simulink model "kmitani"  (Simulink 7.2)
settings: Solver=ode45  StartTime=0.0  StopTime=50  RelTol=1e-3
InitFcn:
  | init_kmitani;
StopFcn:
  | post;
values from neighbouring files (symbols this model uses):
  amp = 5    [init_kmitani.m]
  freq = 50.2248    [init_kmitani.m]
  I_tycka = (m_tycka*l_tycka^2)/12 * [0 0 0;0 1 0; 0 0 1]    [init_kmitani.m]
  I_zavazi = [(m_zavazi/4)*(R_zavazi^2 + (h_zavazi^2)/3 ) 0 0    [init_kmitani.m]
  l_tycka = 1    [init_kmitani.m]
  m = 1    [smykadlo_init.m]
  m_tycka = 0.001    [init_kmitani.m]
  m_zavazi = 10    [init_kmitani.m]
  R_zavazi = 0.1    [init_kmitani.m]
  vule_H = 0.01    [init_kmitani.m]
  vule_L = -0.18    [init_kmitani.m]
undefined symbols (not defined in the file or in its folder): deg, kg, N, s
libraries: mblibv1 x13

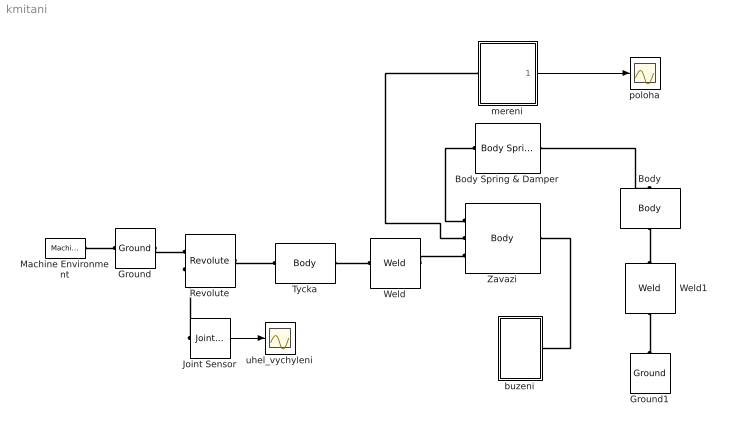
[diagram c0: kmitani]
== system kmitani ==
  Body : mblibv1/Bodies/Body  Orientation=up  DialogController=MECH.DynMechDlgSource  PhysicalDomain=mechanical  SubClassName=Unknown  LeftPortType=workingframe  RightPortType=workingframe  LConnTagsString=CS1  RConnTagsString=CS2  UpdateFromCAD=off  DialogClass=MechanicalBodyBlock  Mass=0  MassUnits=kg  InertiaUnits=kg*m^2  Inertia=zeros(3)  Shape=Cylinder  ShapeDims=[1 1]  ShapeUnits=m  ShapeUse=false  Density=1  DensityUnits=kg/m^3  DensityUse=false  GraphicsMode=MACHINE_DEFAULT  BodyColorSelMode=MACHINE_DEFAULT  BodyColor=[1 0 0]  AttachedToCS=CG  CG=Left$CG$[0 0 0]$CS1$CS1$m$[0 0 0]$Euler X-Y-Z$deg$WORLD$false$none  WorkingFrames=Left$CS1$[0 0 0]$Adjoining$Adjoining$m$[0 0 0]$Euler X-Y-Z$deg$WORLD$true$none#Right$CS2$[0 0 0]$CS1$CS1$m$[0 0 0]$Euler X-Y-Z$deg$WORLD$true$none  CGPos=[0 0 0]  CGRot=[0 0 0]  CS0Pos=[]  CS0Rot=[]  CS1Pos=[0 0 0]  CS1Rot=[0 0 0]  CS2Pos=[0 0 0]  CS2Rot=[0 0 0]  CS3Pos=[]  CS3Rot=[]  CS4Pos=[]  CS4Rot=[]  CS5Pos=[]  CS5Rot=[]  CS6Pos=[]  CS6Rot=[]  CS7Pos=[]  CS7Rot=[]  CS8Pos=[]  CS8Rot=[]  CS9Pos=[]  CS9Rot=[]  CS10Pos=[]  CS10Rot=[]  CS11Pos=[]  CS11Rot=[]  CS12Pos=[]  CS12Rot=[]  CS13Pos=[]  CS13Rot=[]  CS14Pos=[]  CS14Rot=[]  CS15Pos=[]  CS15Rot=[]  CS16Pos=[]  CS16Rot=[]  CS17Pos=[]  CS17Rot=[]  CS18Pos=[]  CS18Rot=[]  CS19Pos=[]  CS19Rot=[]  CS20Pos=[]  CS20Rot=[]
  Body Spring & Damper : mblibv1/Force  Elements/Body Spring & Damper  DialogController=MECH.DynMechDlgSource  SystemSampleTime=-1  UpdateFromCAD=off  DialogClass=BodySpringDamper  Spring_k=k  Damper_b=b  Offset_x0=0  PositionUnits=m  VelocityUnits=m/s  ForceUnits=N
  Ground : mblibv1/Bodies/Ground  DialogController=MECH.DynMechDlgSource  SystemSampleTime=-1  UpdateFromCAD=off  LeftPortType=env  RightPortType=workingframe  PhysicalDomain=Mechanical  DialogClass=GroundBlock  CoordPosition=[0 0 0]  CoordPositionUnits=m  StateVectorMgrId=-1  MachineId=[0 0]  ShowEnvPort=on
  Ground1 : mblibv1/Bodies/Ground  Orientation=up  DialogController=MECH.DynMechDlgSource  SystemSampleTime=-1  UpdateFromCAD=off  LeftPortType=env  RightPortType=workingframe  PhysicalDomain=Mechanical  DialogClass=GroundBlock  CoordPosition=[l_tycka+R_zavazi 0 0]  CoordPositionUnits=m  StateVectorMgrId=-1  MachineId=[0 0]  ShowEnvPort=off
  Joint Sensor : mblibv1/Sensors &  Actuators/Joint Sensor  DialogController=MECH.DynMechDlgSource  SystemSampleTime=-1  UpdateFromCAD=off  PhysicalDomain=Mechanical  PortType=blob  Muxed=on  Pose=off  Angle=on  AngleUnits=rad  ArcVelocity=off  ArcVelocityUnits=deg/s  ArcAcceleration=off  ArcAccelerationUnits=deg/s^2  CoordPosition=on  CoordPositionUnits=m  Velocity=off  VelocityUnits=m/s  Acceleration=off  AccelerationUnits=m/s^2  Quaternion=on  QuaternionDT=off  QuaternionDDT=off  QuaternionUnits=off  OutputVector=[1]  ActiveIO=off  Width=1  DialogClass=MechanicalSensorBlock  Primitive=R1  Force=off  ForceUnits=N  Torque=off  TorqueUnits=N*m  ReferenceFrame=Absolute (World)  ReactionSensedSide=Base  ReactionReferenceFrame=Absolute (World)  ReactionForce=off  ReactionForceUnits=N  ReactionMoment=off  ReactionMomentUnits=N*m
  Machine Environment : mblibv1/Bodies/Machine Environment  DialogController=MECH.DialogSource  SystemSampleTime=-1  PortType=env  PhysicalDomain=Mechanical  DialogTemplateClass=MECH.MachineEnvironment  SyncWhenCopied=off  Gravity=[0 0 0]  GravityUnits=m/s^2  GravityAsSignal=off  Dimensionality=Auto-detect  AnalysisType=Forward dynamics  LinearAssemblyTolerance=1e-3  LinearAssemblyToleranceUnits=m  AngularAssemblyTolerance=1e-3  AngularAssemblyToleranceUnits=rad  ConstraintSolverType=Stabilizing  ConstraintRelTolerance=1e-4  ConstraintAbsTolerance=1e-4  UseRobustSingularityHandling=off  RedundancyAnalysisToleranceType=Automatically select tolerance  RedundancyAnalysisTolerance=1e-14  StatePerturbationType=Fixed  PerturbationSize=1e-5  VisualizeMachine=on  BodyVisualizationType=Use model default body geometries  BodyColorSelMode=Use model default  DefaultBodyColor=[1 0 0]
  Revolute : mblibv1/Joints/Revolute  DialogController=MECH.DynMechDlgSource  PhysicalDomain=mechanical  SubClassName=Unknown  LeftPortType=blob  RightPortType=blob  LConnTagsString=__newl0|SA1  RConnTagsString=__newr0  UpdateFromCAD=off  NumSAPorts=1  CutJoint=off  MarkAsCut=off  Primitives=prismatic  PrimitiveProps=R1$World$[0 0 1]$revolute  DialogClass=JointBlock  R1Axis=[0 0 1]
  Tycka : mblibv1/Bodies/Body  DialogController=MECH.DynMechDlgSource  PhysicalDomain=mechanical  SubClassName=Unknown  LeftPortType=workingframe  RightPortType=workingframe  LConnTagsString=CS1  RConnTagsString=CS2  UpdateFromCAD=off  DialogClass=MechanicalBodyBlock  Mass=m_tycka  MassUnits=kg  InertiaUnits=kg*m^2  Inertia=I_tycka  Shape=Cylinder  ShapeDims=[1 1]  ShapeUnits=m  ShapeUse=false  Density=1  DensityUnits=kg/m^3  DensityUse=false  GraphicsMode=MACHINE_DEFAULT  BodyColorSelMode=MACHINE_DEFAULT  BodyColor=[1 0 0]  AttachedToCS=CG  CG=Left$CG$[l_tycka/2 0 0]$CS1$CS1$m$[0 0 0]$Euler X-Y-Z$deg$WORLD$false$none  WorkingFrames=Left$CS1$[0 0 0]$Adjoining$Adjoining$m$[0 0 0]$Euler X-Y-Z$deg$WORLD$true$none#Right$CS2$[l_tycka 0 0]$CS1$CS1$m$[0 0 0]$Euler X-Y-Z$deg$WORLD$true$none  CGPos=[l_tycka/2 0 0]  CGRot=[0 0 0]  CS0Pos=[]  CS0Rot=[]  CS1Pos=[0 0 0]  CS1Rot=[0 0 0]  CS2Pos=[l_tycka 0 0]  CS2Rot=[0 0 0]  CS3Pos=[]  CS3Rot=[]  CS4Pos=[]  CS4Rot=[]  CS5Pos=[]  CS5Rot=[]  CS6Pos=[]  CS6Rot=[]  CS7Pos=[]  CS7Rot=[]  CS8Pos=[]  CS8Rot=[]  CS9Pos=[]  CS9Rot=[]  CS10Pos=[]  CS10Rot=[]  CS11Pos=[]  CS11Rot=[]  CS12Pos=[]  CS12Rot=[]  CS13Pos=[]  CS13Rot=[]  CS14Pos=[]  CS14Rot=[]  CS15Pos=[]  CS15Rot=[]  CS16Pos=[]  CS16Rot=[]  CS17Pos=[]  CS17Rot=[]  CS18Pos=[]  CS18Rot=[]  CS19Pos=[]  CS19Rot=[]  CS20Pos=[]  CS20Rot=[]
  Weld : mblibv1/Joints/Weld  DialogController=MECH.DynMechDlgSource  PhysicalDomain=mechanical  SubClassName=Unknown  LeftPortType=blob  RightPortType=blob  LConnTagsString=__newl0  RConnTagsString=__newr0  UpdateFromCAD=off  NumSAPorts=0  CutJoint=off  MarkAsCut=off  Primitives=weld  PrimitiveProps=W$WORLD$[0 0 0]$weld  DialogClass=JointBlock  WAxis=[0 0 0]
  Weld1 : mblibv1/Joints/Weld  Orientation=up  DialogController=MECH.DynMechDlgSource  PhysicalDomain=mechanical  SubClassName=Unknown  LeftPortType=blob  RightPortType=blob  LConnTagsString=__newl0  RConnTagsString=__newr0  UpdateFromCAD=off  NumSAPorts=0  CutJoint=off  MarkAsCut=off  Primitives=weld  PrimitiveProps=W$WORLD$[0 0 0]$weld  DialogClass=JointBlock  WAxis=[0 0 0]
  Zavazi : mblibv1/Bodies/Body  DialogController=MECH.DynMechDlgSource  PhysicalDomain=mechanical  SubClassName=Unknown  LeftPortType=workingframe  RightPortType=workingframe  LConnTagsString=CG|CS5|CS1  RConnTagsString=CS2  UpdateFromCAD=off  DialogClass=MechanicalBodyBlock  Mass=m_zavazi  MassUnits=kg  InertiaUnits=kg*m^2  Inertia=I_zavazi  Shape=Cylinder  ShapeDims=[1 1]  ShapeUnits=m  ShapeUse=false  Density=1  DensityUnits=kg/m^3  DensityUse=false  GraphicsMode=MACHINE_DEFAULT  BodyColorSelMode=MACHINE_DEFAULT  BodyColor=[1 0 0]  AttachedToCS=CG  CG=Left$CG$[R_zavazi 0 0]$CS1$CS1$m$[0 0 0]$Euler X-Y-Z$deg$WORLD$true$none  WorkingFrames=Left$CS5$[R_zavazi 0 0]$CS1$CS1$m$[0 0 0]$Euler X-Y-Z$deg$WORLD$true$none#Left$CS1$[0 0 0]$Adjoining$Adjoining$m$[0 0 0]$Euler X-Y-Z$deg$WORLD$true$none#Right$CS2$[R_zavazi*2 0 0]$CS1$CS1$m$[0 0 0]$Euler X-Y-Z$deg$WORLD$true$none#Right$CS3$[R_zavazi R_zavazi 0]$CS1$CS1$m$[0 0 0]$Euler X-Y-Z$deg$WORLD$false$none#Right$CS4$[R_zavazi -R_zavazi 0]$CS1$CS1$m$[0 0 0]$Euler X-Y-Z$deg$WORLD$false$none  CGPos=[R_zavazi 0 0]  CGRot=[0 0 0]  CS0Pos=[]  CS0Rot=[]  CS1Pos=[0 0 0]  CS1Rot=[0 0 0]  CS2Pos=[R_zavazi*2 0 0]  CS2Rot=[0 0 0]  CS3Pos=[R_zavazi R_zavazi 0]  CS3Rot=[0 0 0]  CS4Pos=[R_zavazi -R_zavazi 0]  CS4Rot=[0 0 0]  CS5Pos=[R_zavazi 0 0]  CS5Rot=[0 0 0]  CS6Pos=[]  CS6Rot=[]  CS7Pos=[]  CS7Rot=[]  CS8Pos=[]  CS8Rot=[]  CS9Pos=[]  CS9Rot=[]  CS10Pos=[]  CS10Rot=[]  CS11Pos=[]  CS11Rot=[]  CS12Pos=[]  CS12Rot=[]  CS13Pos=[]  CS13Rot=[]  CS14Pos=[]  CS14Rot=[]  CS15Pos=[]  CS15Rot=[]  CS16Pos=[]  CS16Rot=[]  CS17Pos=[]  CS17Rot=[]  CS18Pos=[]  CS18Rot=[]  CS19Pos=[]  CS19Rot=[]  CS20Pos=[]  CS20Rot=[]
  buzeni : Subsystem
  mereni : Subsystem
  poloha : Scope
  uhel_vychyleni : Scope
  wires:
  mereni/1(Out1) -> poloha/1
  Joint Sensor/1 -> uhel_vychyleni/1
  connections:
  Machine Environment/RConn1 -- Ground/LConn1
  Ground/RConn1 -- Revolute/LConn1
  Revolute/RConn1 -- Tycka/LConn1
  Tycka/RConn1 -- Weld/LConn1
  Weld/RConn1 -- Zavazi/LConn3
  Ground1/RConn1 -- Weld1/LConn1
  Weld1/RConn1 -- Body/LConn1
  Zavazi/LConn1 -- Body Spring & Damper/LConn1
  Body Spring & Damper/RConn1 -- Body/RConn1
  buzeni/RConn1 -- Zavazi/RConn1
  Zavazi/LConn2 -- mereni/LConn1
  Joint Sensor/LConn1 -- Revolute/LConn2

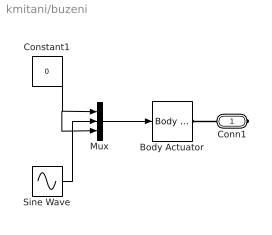
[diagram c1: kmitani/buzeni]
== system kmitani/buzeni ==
  Body Actuator : mblibv1/Sensors &  Actuators/Body Actuator  DialogController=MECH.DynMechDlgSource  SystemSampleTime=-1  UpdateFromCAD=off  PhysicalDomain=Mechanical  PortType=blob  ActuationStyle=Force  AngleUnits=deg  ArcVelocityUnits=deg/s  ArcAccelerationUnits=deg/s^2  CoordPositionUnits=m  VelocityUnits=m/s  AccelerationUnits=m/s^2  ForceUnits=N  TorqueUnits=N*m  ActiveIO=off  Width=3  DialogClass=MechanicalActuatorBlock  ReferenceFrame=Local (Body CS)  Angle=off  CoordPosition=on  Force=on  Torque=off
  Constant1 : Constant  Value=0  OutDataType=fixdt(1, 16)  OutScaling=2^0
  Mux : Mux  Inputs=3
  Sine Wave : Sin  Amplitude=amp  Frequency=freq*2*pi  SampleTime=0
  Conn1 : PMIOPort  Orientation=left  Port=1  Side=Right
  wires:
  Mux/1 -> Body Actuator/1
  Constant1/1 -> Mux/1, Mux/3
  Sine Wave/1 -> Mux/2
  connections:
  Conn1/RConn1 -- Body Actuator/RConn1

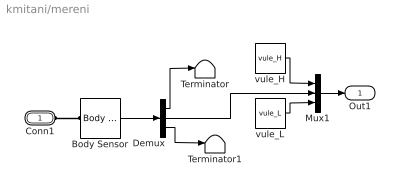
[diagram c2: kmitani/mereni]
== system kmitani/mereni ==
  Body Sensor : mblibv1/Sensors &  Actuators/Body Sensor  DialogController=MECH.DynMechDlgSource  SystemSampleTime=-1  UpdateFromCAD=off  PhysicalDomain=Mechanical  PortType=blob  Muxed=on  Pose=off  Angle=on  AngleUnits=deg  ArcVelocity=off  ArcVelocityUnits=deg/s  ArcAcceleration=off  ArcAccelerationUnits=deg/s^2  CoordPosition=on  CoordPositionUnits=m  Velocity=off  VelocityUnits=m/s  Acceleration=off  AccelerationUnits=m/s^2  Quaternion=on  QuaternionDT=off  QuaternionDDT=off  QuaternionUnits=off  OutputVector=[1]  ActiveIO=off  Width=3  DialogClass=MechanicalSensorBlock  ReferenceFrame=Absolute (World)
  Demux : Demux  Outputs=3
  Mux1 : Mux  Inputs=3
  Terminator : Terminator
  Terminator1 : Terminator
  vule_H : Constant  Value=vule_H  OutDataType=fixdt(1, 16)  OutScaling=2^0
  vule_L : Constant  Value=vule_L  OutDataType=fixdt(1, 16)  OutScaling=2^0
  Conn1 : PMIOPort  Port=1  Side=Left
  Out1 : Outport
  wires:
  Body Sensor/1 -> Demux/1
  Demux/1 -> Terminator/1
  Demux/3 -> Terminator1/1
  vule_H/1 -> Mux1/1
  Demux/2 -> Mux1/2
  vule_L/1 -> Mux1/3
  Mux1/1 -> Out1/1
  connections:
  Conn1/RConn1 -- Body Sensor/LConn1
